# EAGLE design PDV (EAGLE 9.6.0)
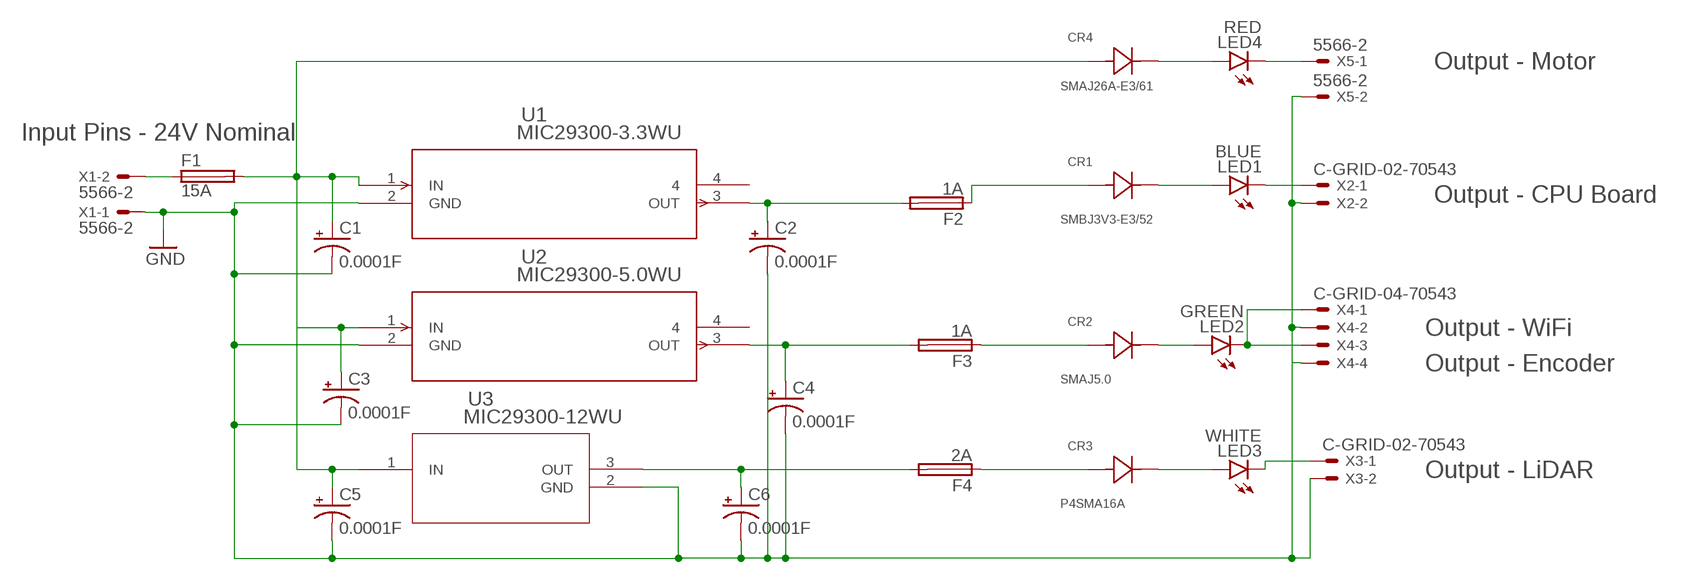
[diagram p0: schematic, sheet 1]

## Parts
C1  0.0001F  CPOL-USE2.5-6  [E2,5-6]
C2  0.0001F  CPOL-USE2.5-6  [E2,5-6]
C3  0.0001F  CPOL-USE2.5-6  [E2,5-6]
C4  0.0001F  CPOL-USE2.5-6  [E2,5-6]
C5  0.0001F  CPOL-USE2.5-6  [E2,5-6]
C6  0.0001F  CPOL-USE2.5-6  [E2,5-6]
CR1  SMBJ3V3-E3/52  [CR_V3-E3/52_VIS]
CR2  SMAJ5.0  [SMASERIES_LTF]
CR3  P4SMA16A  [P4SMASERIES_LTF]
CR4  SMAJ26A-E3/61  [DIODE_DO-214AC]
F1  15A  TE5  [TE5]
F2  1A  TE5  [TE5]
F3  1A  TE5  [TE5]
F4  2A  TE5  [TE5]
LED1  BLUE  LEDSMT1206  [1206]
LED2  GREEN  LEDSMT1206  [1206]
LED3  WHITE  LEDSMT1206  [1206]
LED4  RED  LEDSMT1206  [1206]
U1  MIC29300-3.3WU  [TO-263-3_MCL]
U2  MIC29300-5.0WU  [TO-263-3_MCL]
U3  MIC29300-12WU  [TO220-3LD-PL-1_MCH]
X1  5566-2  [5566-2]
X2  C-GRID-02-70543  [70543-02]
X3  C-GRID-02-70543  [70543-02]
X4  C-GRID-04-70543  [70543-04]
X5  5566-2  [5566-2]

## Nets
GND: C1.- C2.- C3.- C4.- C5.- C6.- U1.2(GND) U2.2(GND) U3.2(GND) X1.1 X2.2 X3.2 X4.2 X4.4 X5.2
N$1: F1.1 X1.2
N$2: C1.+ C3.+ C5.+ CR4.2 F1.2 U1.1(IN) U2.1(IN) U3.1(IN)
N$3: C2.+ F2.2 U1.3(OUT)
N$4: C4.+ F3.2 U2.3(OUT)
N$5: C6.+ F4.2 U3.3(OUT)
N$7: CR1.2 F2.1
N$8: CR2.2 F3.1
N$9: CR3.2 F4.1
N$13: CR4.1 LED4.A
N$14: LED4.C X5.1
N$15: CR1.1 LED1.A
N$16: LED1.C X2.1
N$17: CR2.1 LED2.A
N$18: LED2.C X4.1 X4.3
N$19: CR3.1 LED3.A
N$20: LED3.C X3.1
Unconnected: U1.4 U2.4

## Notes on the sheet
- Output - Motor
- Input Pins - 24V Nominal
- Output - CPU Board
- Output - WiFi
- Output - Encoder
- Output - LiDAR

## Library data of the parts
C1-C6 = rcl:CPOL-US: POLARIZED CAPACITOR, American symbol; SPICEPREFIX: C
CR1 = SMBJ3V3-E3:SMBJ3V3-E3/52; COPYRIGHT: Copyright (C) 2025 Ultra Librarian. All rights reserved.; MANUFACTURER_PART_NUMBER: SMBJ3V3-E3/52; MFR_NAME: Vishay
CR2 = SMAJ5.0:SMAJ5.0; COPYRIGHT: Copyright (C) 2025 Ultra Librarian. All rights reserved.; MANUFACTURER_PART_NUMBER: SMAJ5.0; MFR_NAME: Littelfuse Inc
CR3 = P4SMA16A:P4SMA16A; COPYRIGHT: Copyright (C) 2025 Ultra Librarian. All rights reserved.; MANUFACTURER_PART_NUMBER: P4SMA16A; MFR_NAME: Littelfuse Inc
CR4 = SMAJ26A-E3:SMAJ26A-E3/61; COPYRIGHT: Copyright (C) 2025 Ultra Librarian. All rights reserved.; MANUFACTURER_PART_NUMBER: SMAJ26A-E3/61; MFR_NAME: Vishay
F1-F4 = fuse:TE5: FUSE; OC_FARNELL: unknown; OC_NEWARK: unknown
LED1-LED4 = led:LED: LED
U1 = MIC29300-3.3:MIC29300-3.3WU; COPYRIGHT: Copyright (C) 2025 Ultra Librarian. All rights reserved.; MANUFACTURER_PART_NUMBER: MIC29300-3.3WU; MFR_NAME: Micrel / Microchip Technology
U2 = MIC29300-5.0lbr:MIC29300-5.0WU; COPYRIGHT: Copyright (C) 2025 Ultra Librarian. All rights reserved.; MANUFACTURER_PART_NUMBER: MIC29300-5.0WU; MFR_NAME: Micrel / Microchip Technology
U3 = MIC29300-12:MIC29300-12WU; COPYRIGHT: Copyright (C) 2025 Ultra Librarian. All rights reserved.; MANUFACTURER_PART_NUMBER: MIC29300-12WU; MFR_NAME: Micrel / Microchip Technology
X1 X5 = con-molex:5566-2: Mini FIT connector 2 pol; MF: MOLEX; OC_FARNELL: 1822072; OC_NEWARK: unknown
X2 X3 = con-molex:C-GRID-02: CONNECTOR; MF: MOLEX; OC_FARNELL: unknown; OC_NEWARK: unknown
X4 = con-molex:C-GRID-04: CONNECTOR wire to board 2.54 mm (0.100") pitch header; MF: MOLEX; OC_FARNELL: unknown; OC_NEWARK: unknown

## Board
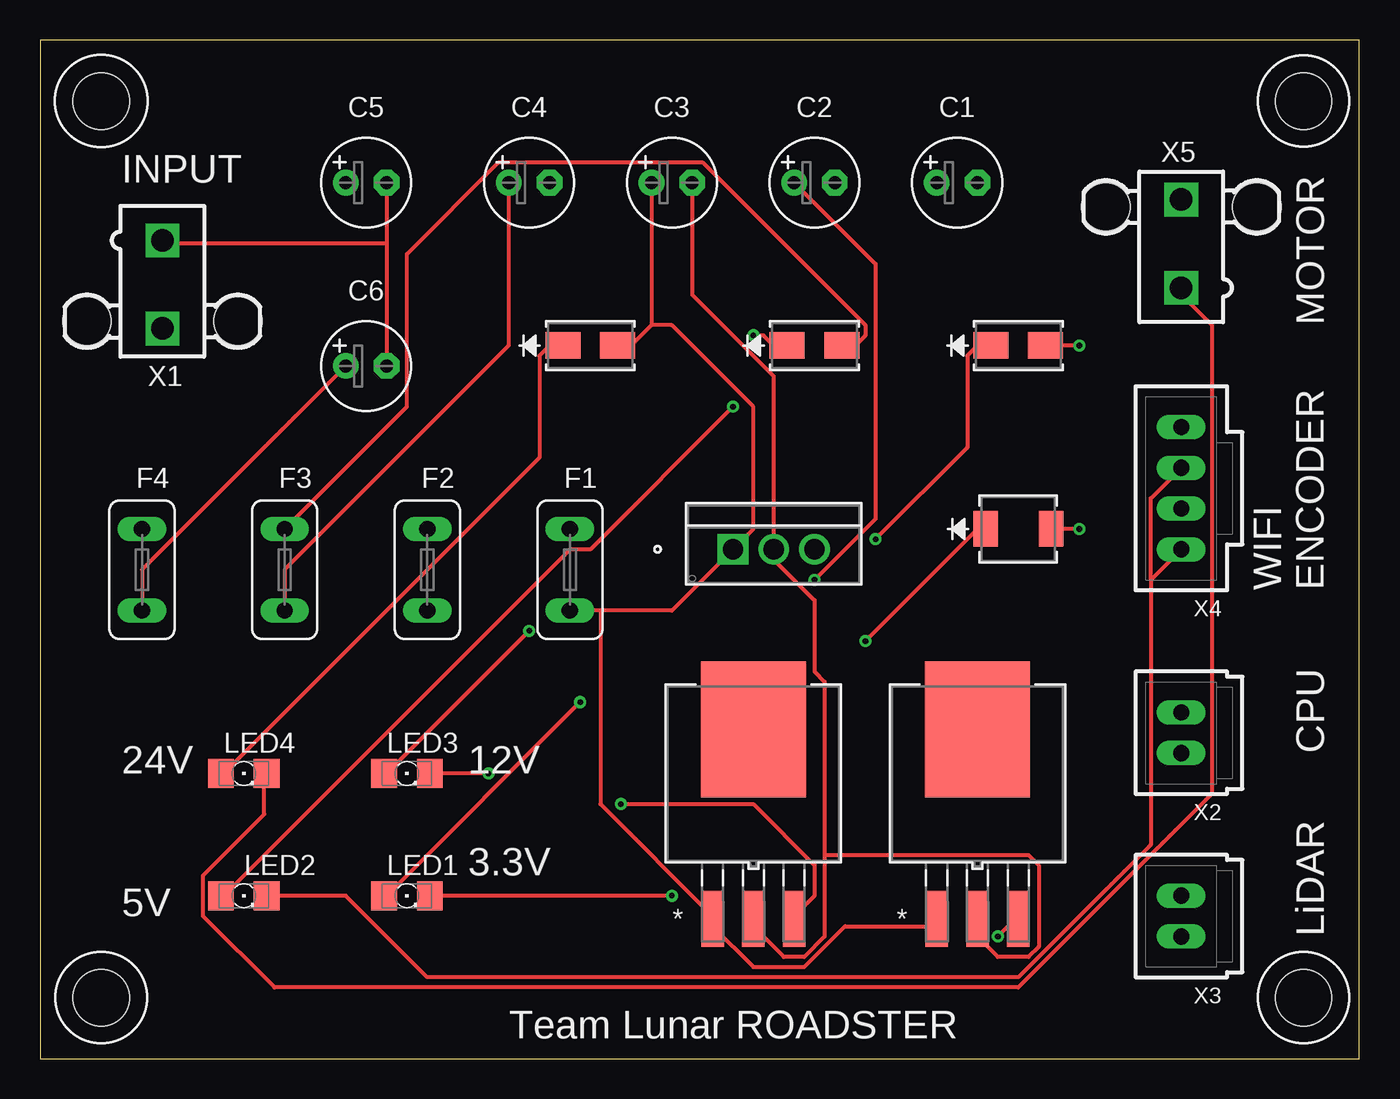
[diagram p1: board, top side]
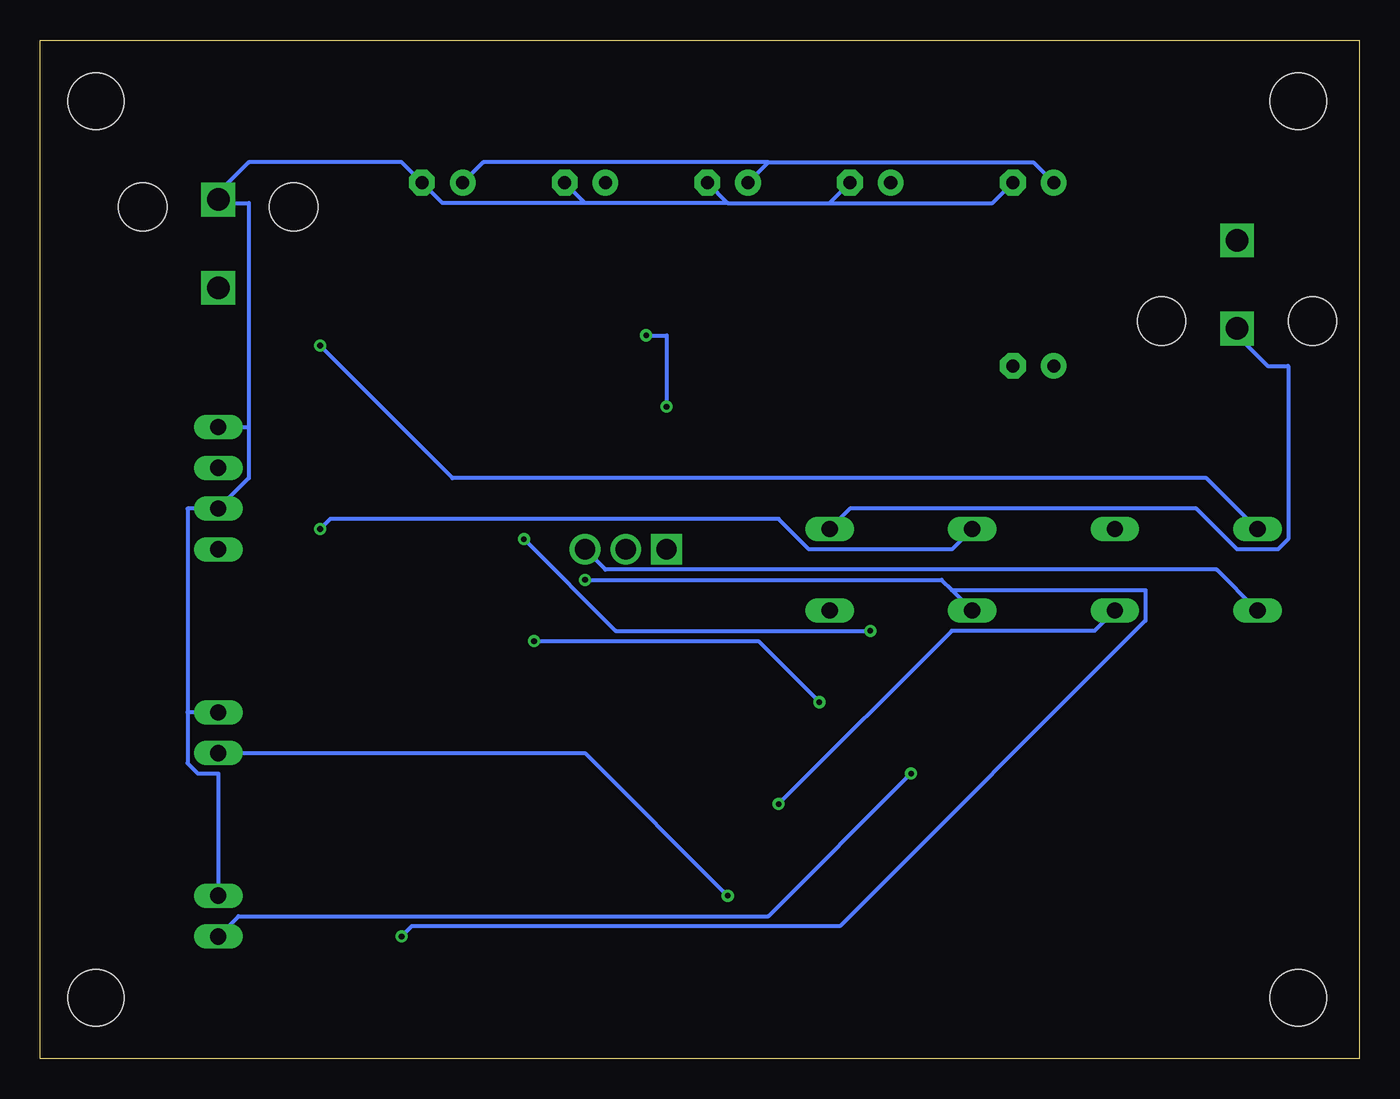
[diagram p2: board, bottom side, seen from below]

Size 82.22 x 63.49 mm. Coordinates in mm from the lower left corner, seen from the top.
Outline: 0,0 82.22,0 82.22,63.49 0,63.49 0,0
Copper layers (1*16): Top 0.035mm / dielectric 1.5mm / Bottom 0.035mm
Design rules "default *": minimum track width 10mil, minimum drill 0.35mm, track to track 6mil, track to pad 6mil, pad to pad 6mil, via to via 6mil, smd to smd 6mil, copper to edge 40mil, drill to drill 6mil, minimum pad ring 10mil, minimum via ring 8mil, stop-mask expansion 4mil, vias tented up to drill 0mil, thermal gap 10mil
Holes 3.51 mm at 3.81,59.69 78.74,59.69 78.74,3.81 3.81,3.81

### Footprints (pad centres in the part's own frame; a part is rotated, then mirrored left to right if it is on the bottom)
E2,5-6 = drill 0.813 pad 1.6: + -1.27,0 | drill 0.813 pad 1.6 octagon: - 1.27,0
CR_V3-E3/52_VIS = smd 1.524 x 2.21: 1 -2.035,0; 2 2.035,0
SMASERIES_LTF = smd 2.184 x 1.651: 1 -1.702,0; 2 1.702,0
P4SMASERIES_LTF = smd 2.184 x 1.651: 1 -1.702,0; 2 1.702,0
DIODE_DO-214AC = smd 2.184 x 1.651: 1 -1.702,0; 2 1.702,0
TE5 = drill 1.016 long: 1 -2.54,0; 2 2.54,0
1206 = smd 1.6 x 1.803: A -1.422,0; C 1.422,0
TO-263-3_MCL = smd 1.397 x 3.505: 1 -2.54,-9.055; 2 0,-9.055; 3 2.54,-9.055 | smd 6.553 x 8.458: 4 0,2.743
TO220-3LD-PL-1_MCH = drill 1.27 pad 1.778 square: 1 0,0 | drill 1.27 pad 1.778: 2 2.54,0; 3 5.08,0
5566-2 = drill 1.4 square: 1 0,-2.75; 2 0,2.75 | hole 3: 4.7,2.29; -4.7,2.29
70543-02 = drill 1.016 long: 1 -1.27,0; 2 1.27,0
70543-04 = drill 1.016 long: 1 -3.81,0; 2 -1.27,0; 3 1.27,0; 4 3.81,0

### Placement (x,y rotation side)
C1  57.15,54.61 0 top
C2  48.26,54.61 0 top
C3  39.37,54.61 0 top
C4  30.48,54.61 0 top
C5  20.32,54.61 0 top
C6  20.32,43.18 0 top
CR1  60.96,33.02 0 top
CR2  48.26,44.45 0 top
CR3  60.96,44.45 0 top
CR4  34.29,44.45 0 top
F1  33.02,30.48 270 top
F2  24.13,30.48 270 top
F3  15.24,30.48 270 top
F4  6.35,30.48 270 top
LED1  22.86,10.16 0 top
LED2  12.7,10.16 0 top
LED3  22.86,17.78 0 top
LED4  12.7,17.78 0 top
U1  58.42,17.78 0 top
U2  44.45,17.78 0 top
U3  43.18,31.75 0 top
X1  7.62,48.26 180 top
X2  71.12,20.32 90 top
X3  71.12,8.89 90 top
X4  71.12,35.56 90 top
X5  71.12,50.8 0 top

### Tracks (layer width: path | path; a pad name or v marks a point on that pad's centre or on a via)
GND
  Top 0.254: 48.89,12.7 48.89,23.5 48.26,24.13 48.26,28.58 45.72,31.12 U3.2 45.72,42.55 40.64,47.62 C3.- | 48.89,12.7 48.89,7.62 47.62,6.35 46.36,6.35 44.45,8.26 U2.2 | U1.2 58.42,7.62 59.69,6.35 61.59,6.35 62.23,6.98 62.23,12.06 61.59,12.7 48.89,12.7 | C5.- 21.59,50.8 | 21.59,50.8 C6.- | 21.59,50.8 7.62,50.8 X1.1
  Bottom 0.254: X3.2 71.12,17.78 72.39,17.78 73.03,18.41 73.03,21.59 | X2.2 73.03,21.59 | 69.22,39.37 69.22,36.2 X4.2 73.03,34.29 73.03,21.59 | X4.4 69.22,39.37 | 33.02,53.34 C4.- | 39.37,53.34 33.02,53.34 | C3.- 39.37,53.34 | 48.26,53.34 C2.- | 39.37,53.34 48.26,53.34 | 48.26,53.34 57.15,53.34 C1.- 59.69,55.88 69.22,55.88 71.12,53.97 X5.2 71.12,53.34 69.22,53.34 69.22,39.37 | C5.- 22.86,53.34 33.02,53.34
N$1
  Bottom 0.254: F1.1 31.75,34.29 10.16,34.29 7.62,31.75 5.08,31.75 4.45,32.38 4.45,43.18 5.71,43.18 7.62,45.09 X1.2
N$2
  Top 0.254: CR4.2 36.83,44.45 38.1,45.72 | C3.+ 38.1,45.72 | 34.92,27.94 39.37,27.94 U3.1 44.45,33.02 44.45,40.64 39.37,45.72 38.1,45.72 | 34.92,27.94 F1.2 | 34.92,27.94 34.92,15.87 41.91,8.89 U2.1 41.91,8.26 44.45,5.71 47.62,5.71 50.16,8.26 55.88,8.26 U1.1
  Bottom 0.254: C5.+ 20.32,55.88 36.83,55.88 | C3.+ 36.83,55.88 | C1.+ 54.61,55.88 36.83,55.88
N$3  (via drill 0.35)
  Top 0.254: v48.26,29.84 52.07,33.66 52.07,49.53 C2.+ | v59.69,7.62 60.33,8.26 60.96,8.26 U1.3
  Bottom 0.254: 25.4,29.21 26.03,29.84 v48.26,29.84 | 25.4,29.21 F2.2 | v59.69,7.62 59.05,8.26 32.38,8.26 13.33,27.3 13.33,29.21 25.4,29.21
N$4  (via drill 0.35)
  Top 0.254: F3.2 15.24,30.48 29.21,44.45 C4.+ | v36.2,15.87 44.45,15.87 48.26,12.06 48.26,10.16 46.99,8.89 U2.3
  Bottom 0.254: v36.2,15.87 25.4,26.67 16.51,26.67 F3.2
N$5
  Top 0.254: F4.2 6.35,30.48 C6.+
  Bottom 0.254: U3.3 46.99,30.48 8.89,30.48 F4.2
N$7  (via drill 0.35)
  Top 0.254: v64.77,33.02 CR1.2
  Bottom 0.254: v64.77,33.02 64.14,33.66 36.2,33.66 34.29,31.75 25.4,31.75 F2.1
N$8
  Top 0.254: CR2.2 50.8,44.45 51.44,45.09 51.44,45.72 41.27,55.88 28.57,55.88 22.86,50.17 22.86,40.64 F3.1
N$9  (via drill 0.35)
  Top 0.254: v64.77,44.45 CR3.2
  Bottom 0.254: v64.77,44.45 56.52,36.2 9.52,36.2 F4.1
N$13
  Top 0.254: CR4.1 31.75,44.45 31.12,43.81 31.12,37.47 11.43,17.78 LED4.A
N$14
  Top 0.254: LED4.C 13.97,17.78 13.97,15.24 10.16,11.43 10.16,8.89 14.6,4.44 60.96,4.44 73.03,16.51 73.03,45.72 71.12,47.62 X5.1
N$15  (via drill 0.35)
  Top 0.254: v33.66,22.23 21.59,10.16 LED1.A | v51.44,26.04 58.42,33.02 CR1.1
  Bottom 0.254: v33.66,22.23 37.46,26.04 v51.44,26.04
N$16  (via drill 0.35)
  Top 0.254: v39.37,10.16 LED1.C
  Bottom 0.254: v39.37,10.16 48.26,19.05 X2.1
N$17  (via drill 0.35)
  Top 0.254: v43.18,40.64 34.29,31.75 33.02,31.75 11.43,10.16 LED2.A | v44.45,45.09 45.09,45.09 45.72,44.45 CR2.1
  Bottom 0.254: v43.18,40.64 43.18,45.09 v44.45,45.09
N$18
  Top 0.254: LED2.C 19.05,10.16 24.13,5.08 60.96,5.08 69.22,13.33 69.22,29.84 | X4.1 69.22,29.84 | X4.3 69.22,34.93 69.22,29.84
N$19  (via drill 0.35)
  Top 0.254: v30.48,26.67 21.59,17.78 LED3.A | v52.07,32.38 57.78,38.1 57.78,43.81 58.42,44.45 CR3.1
  Bottom 0.254: v30.48,26.67 46.36,26.67 v52.07,32.38
N$20  (via drill 0.35)
  Top 0.254: v27.94,17.78 LED3.C
  Bottom 0.254: v27.94,17.78 36.83,8.89 69.85,8.89 X3.1

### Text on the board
tNames: INPUT | MOTOR | WIFI / ENCODER | CPU | 24V | 12V | 3.3V | 5V | LiDAR | Team Lunar ROADSTER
